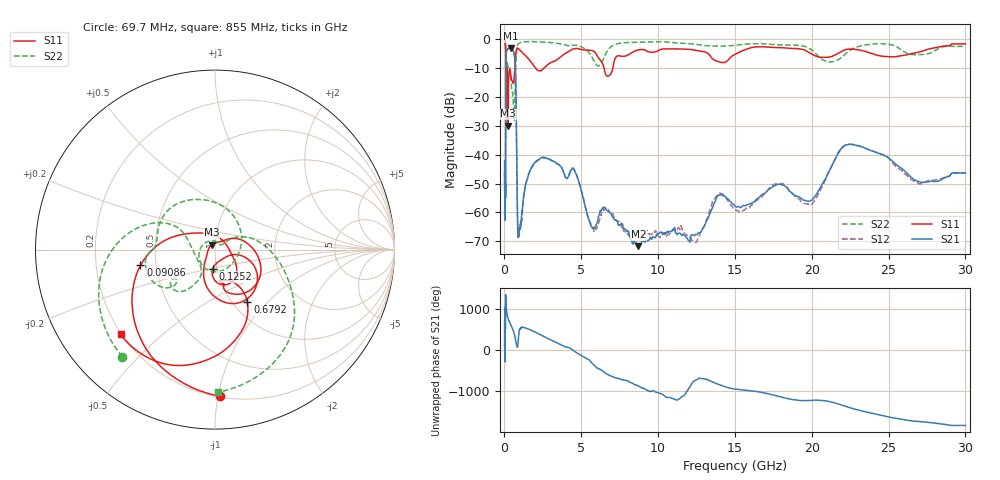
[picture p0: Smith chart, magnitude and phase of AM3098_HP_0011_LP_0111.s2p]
! Date/Time: Thu, Feb 28, 2019 8:34 AM
! Network Analyzer: Agilent Technologies E8364B Rev: A.07.50.67
! Sweep from 0.010 to 30.000 GHz, 1601 Points, Sweep Type: LOG
! Power Supply: 5.022 V, 0.002 A
# Hz S DB R 50
!freq MagS11 AngS11 MagS21 AngS21 MagS12 AngS12 MagS22 AngS22
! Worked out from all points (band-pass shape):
!   1601 points, 10 MHz to 30 GHz, reference 50 ohm
!   highest |S21| = -3.10 dB at 418 MHz (marker M1); lowest = -71.7 dB at 8.716 GHz (marker M2)
!   |S21| within 3 dB of the highest: 107.6 MHz to 660.3 MHz (552.7 MHz wide, 144 % of centre)
!   lowest |S11| = -29.9 dB at 228.2 MHz (marker M3), VSWR 1.07, Z = 48.2 + j2.61 ohm
!   |S11| at or under -10 dB: 176 MHz to 671.3 MHz (495.3 MHz wide, 117 % of centre); 2.04 GHz to 2.551 GHz (511.6 MHz wide, 22.3 % of centre); 6.487 GHz to 7.049 GHz (561.7 MHz wide, 8.3 % of centre)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
!   |S22| runs from -28.3 to -0.6 dB; largest |S21 - S12| = 0.0096
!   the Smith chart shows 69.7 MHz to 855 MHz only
!   S11 on the Smith chart (normalised r, x): 69.7 MHz: 0.21, -1.02; 90.86 MHz: 0.41, -0.09; 125.2 MHz: 0.95, -0.21; 679.2 MHz: 1.16, -0.77; 855 MHz: 0.20, -0.37
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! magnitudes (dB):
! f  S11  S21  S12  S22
! 10 MHz  -0.3  -42.2  -46.1  -0.6
! 38.04 MHz  -0.5  -60.1  -60.8  -0.9
! 69.7 MHz  -1.8  -52.3  -53.6  -2.1
! 90.86 MHz  -7.4  -20.8  -20.8  -8.6
! 100.9 MHz  -23.5  -8.2  -8.2  -16.8
! 125.2 MHz  -19.3  -4.4  -4.4  -10.5
! 144.7 MHz  -14.0  -3.7  -3.7  -10.4
! 184.9 MHz  -11.1  -3.6  -3.6  -8.0
! 228.2 MHz  -29.9  -3.2  -3.2  -9.5
! 418 MHz  -12.5  -3.1  -3.1  -13.2
! 550.5 MHz  -15.1  -3.8  -3.7  -19.3
! 679.2 MHz  -9.3  -7.2  -7.2  -21.6
! 747 MHz  -4.8  -18.0  -17.9  -8.0
! 855 MHz  -3.0  -63.5  -64.1  -2.0
! 2.084 GHz  -10.3  -42.2  -42.2  -0.8
! 4.503 GHz  -3.3  -45.0  -44.8  -2.0
! 5.697 GHz  -3.9  -65.1  -64.9  -6.1
! 7.926 GHz  -5.7  -66.1  -67.2  -1.1
! 8.716 GHz  -3.6  -71.7  -66.9  -1.0
! 19.7 GHz  -4.2  -56.1  -57.1  -2.8
! 22.67 GHz  -3.4  -36.4  -36.5  -3.2
! 30 GHz  -1.5  -46.3  -46.3  -2.4
